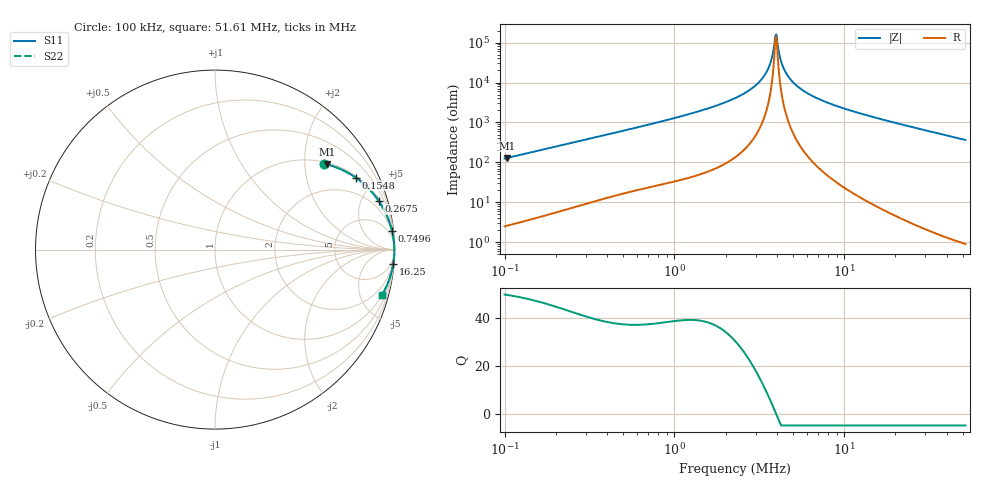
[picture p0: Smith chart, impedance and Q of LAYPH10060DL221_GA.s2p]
! LAYPH10060DL221_GA  S-PARAMETER MODEL  ( General Type )
! Model Generated by TAIYO YUDEN Corporation (http://www.ty-top.com)
! Version 3.0
! TAIYO YUDEN Control No. 180828NI43SB-FBB
! Copyright(c) 2017 TAIYO YUDEN CO.,LTD. All Rights Reserved.
! Product Description (link to TY-COMPAS)
! https://ds.yuden.co.jp/TYCOMPAS/or/detail?pn=LAYPH10060DL221MGA&u=M
! Products Name : Inductors
! Characteristics :
!  Inductance : 220 uH , SRF(min) : -Hz , DC Resistance(max) : 0.384 Ohm
!  Rated Current : Saturation :0.95 A , Temp Rise : 0.66 A (25 degC)
!  Case Size : 10.1 x 10.0 / 0.398 x 0.394 [mm/inch] , Thickness : 6 / 0.236 [mm/inch]
!  (Conditions: Temperature = 25 degC , DC Bias Current/Voltage = 0A / 0V)
! External Node Assignments :
!  1  o---GGG---o  2
! GND o---------o GND
! Frequency Range : 0.1MHz  -  51.610281MHz  [ 402 STEP ]
# MHz S RI R 50
! Freq[MHz].  S11 Real  S11 Imag  S21 Real  S21 Imag  S12 Real  S12 Imag  S22 Real  S22 Imag
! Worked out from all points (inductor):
!   401 points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, 100 kHz to 51.61 MHz, reference 50 ohm
!   read as one part in series: L = 199 uH near 103.2 kHz
!   highest Q = 49.7 at 103.2 kHz (marker M1), where L = 199 uH
!   self-resonance near 3.924 MHz
!   S11 on the Smith chart (normalised r, x): 100 kHz: 1.05, +2.50; 154.8 kHz: 1.08, +3.86; 267.5 kHz: 1.16, +6.65; 749.6 kHz: 2, +19; 16.25 MHz: 1, -25; 51.61 MHz: 1.02, -7.31
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0.1  0.6086 0.4781  0.3914 -0.4781  0.3914 -0.4781  0.6086 0.4781
0.103172  0.6229 0.4747  0.3771 -0.4747  0.3771 -0.4747  0.6229 0.4747
0.154843  0.7838 0.4012  0.2162 -0.4012  0.2162 -0.4012  0.7838 0.4012
0.267458  0.9115 0.2722  0.0885 -0.2722  0.0885 -0.2722  0.9115 0.2722
0.284697  0.9206 0.2585  0.0794 -0.2585  0.0794 -0.2585  0.9206 0.2585
0.749648  0.9862 0.1042  0.0138 -0.1042  0.0138 -0.1042  0.9862 0.1042
0.810525  0.9881 0.0961  0.0119 -0.0961  0.0119 -0.0961  0.9881 0.0961
2.27179  0.9986 0.0246  0.00141 -0.0246  0.00141 -0.0246  0.9986 0.0246
2.826922  0.9991 0.0145  0.000893 -0.0145  0.000893 -0.0145  0.9991 0.0145
3.304702  0.9993 0.00766  0.000679 -0.00766  0.000679 -0.00766  0.9993 0.00766
3.629304  0.9994 0.00368  0.000604 -0.00368  0.000604 -0.00368  0.9994 0.00368
3.863231  0.9994 0.00105  0.000575 -0.00105  0.000575 -0.00105  0.9994 0.00105
3.98579  0.9994 -0.000271  0.000566 0.000271  0.000566 0.000271  0.9994 -0.000271
4.048519  0.9994 -0.000929  0.000563 0.000929  0.000563 0.000929  0.9994 -0.000929
4.309467  0.9994 -0.00357  0.000561 0.00357  0.000561 0.00357  0.9994 -0.00357
4.65943  0.9994 -0.00688  0.000581 0.00688  0.000581 0.00688  0.9994 -0.00688
5.362525  0.9993 -0.013  0.00068 0.013  0.00068 0.013  0.9993 -0.013
6.467723  0.999 -0.0215  0.000955 0.0215  0.000955 0.0215  0.999 -0.0215
9.262618  0.9979 -0.0402  0.00209 0.0402  0.00209 0.0402  0.9979 -0.0402
16.251  0.9929 -0.0809  0.00706 0.0809  0.00706 0.0809  0.9929 -0.0809
18.41343  0.9909 -0.0927  0.00915 0.0927  0.00915 0.0927  0.9909 -0.0927
51.61028  0.9299 -0.2541  0.0701 0.2541  0.0701 0.2541  0.9299 -0.2541
